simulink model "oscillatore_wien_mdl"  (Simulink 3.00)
settings: Solver=ode23s  StartTime=0.0  StopTime=10.0  RelTol=1e-6  AbsTol=1e-6
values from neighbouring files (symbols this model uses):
  beta = 60    [oscillatore.m]    (also in oscillatore_RC.m = 100; oscillatore_wien.m = 3.5)
  C = 0.001    [oscillatore.m]    (also in oscillatore_RC.m; oscillatore_RC_1.m; oscillatore_wien.m)
  Q0 = C*V0    (= 0.0001)    [oscillatore_wien.m]
  R = 1    [oscillatore.m]    (also in oscillatore_RC.m; oscillatore_RC_1.m; oscillatore_wien.m)
  VM = 12    [oscillatore.m]    (also in oscillatore_RC.m; oscillatore_RC_1.m; oscillatore_wien.m)

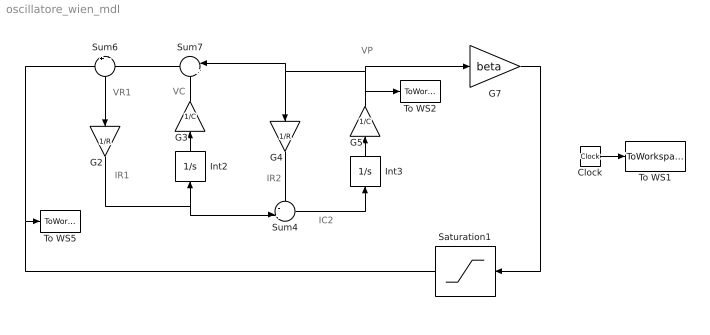
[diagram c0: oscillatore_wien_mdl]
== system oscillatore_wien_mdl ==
  note: VR1
  note: IR1
  note: VC
  note: VP
  note: IR2
  note: IC2
  Clock : Clock
  G2 : Gain  Orientation=down  Gain=1/R  SaturateOnIntegerOverflow=on
  G3 : Gain  Orientation=up  Gain=1/C  SaturateOnIntegerOverflow=on
  G4 : Gain  Orientation=down  Gain=1/R  SaturateOnIntegerOverflow=on
  G5 : Gain  Orientation=up  Gain=1/C  SaturateOnIntegerOverflow=on
  G7 : Gain  Gain=beta  SaturateOnIntegerOverflow=on
  Int2 : Integrator  Orientation=up  ExternalReset=none  InitialConditionSource=internal  InitialCondition=Q0  LimitOutput=off  UpperSaturationLimit=inf  LowerSaturationLimit=-inf  ShowSaturationPort=off  ShowStatePort=off  AbsoluteTolerance=auto
  Int3 : Integrator  Orientation=up  ExternalReset=none  InitialConditionSource=internal  InitialCondition=Q0  LimitOutput=off  UpperSaturationLimit=inf  LowerSaturationLimit=-inf  ShowSaturationPort=off  ShowStatePort=off  AbsoluteTolerance=auto
  Saturation1 : Saturate  Orientation=left  UpperLimit=VM  LowerLimit=-VM
  Sum4 : Sum  Inputs=-+|  SaturateOnIntegerOverflow=on
  Sum6 : Sum  Orientation=down  Inputs=+|-  SaturateOnIntegerOverflow=on
  Sum7 : Sum  Orientation=left  Inputs=|++  SaturateOnIntegerOverflow=on
  To WS1 : ToWorkspace  VariableName=t  SampleTime=-1  SaveFormat=Matrix
  To WS2 : ToWorkspace  VariableName=VP  SampleTime=-1  SaveFormat=Matrix
  To WS5 : ToWorkspace  VariableName=V0  SampleTime=-1  SaveFormat=Matrix
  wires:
  Int2/1 -> G3/1
  Int3/1 -> G5/1
  Sum6/1 -> G2/1
  G3/1 -> Sum7/2
  Sum7/1 -> Sum6/2
  G2/1 -> Int2/1, Sum4/2
  G4/1 -> Sum4/1
  Sum4/1 -> Int3/1
  G5/1 -> To WS2/1, G7/1, Sum7/1, G4/1
  Saturation1/1 -> To WS5/1, Sum6/1
  G7/1 -> Saturation1/1
  Clock/1 -> To WS1/1
